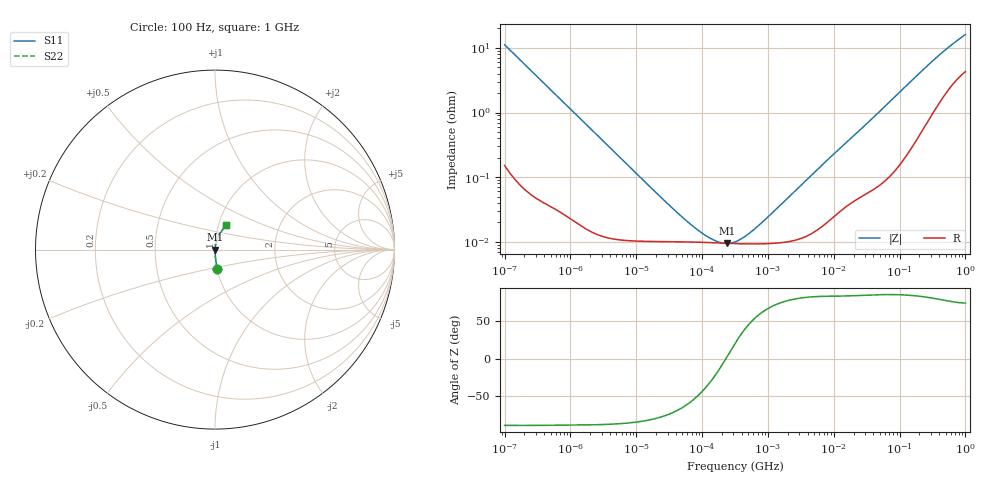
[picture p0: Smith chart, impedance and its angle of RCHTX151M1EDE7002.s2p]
! RCHTX151M1EDE7002  S-PARAMETER MODEL  (AEC-Q200 qualified)
! Model Generated by ELNA Corporation (http://www.ty-top.com)
! Version 1.0
! ELNA Control No.231201
! Copyright (c) 2023 ELNA CO.,LTD. All Rights Reserved.
! Products Name : CONDUCTIVE POLYMER HYBRID ALUMINUM ELECTROLYTIC CAPACITORS
! Characteristics :
!  Capacitance  :  150uF  ,  Rated voltage  :  16V
!  Operating Temp. Range  :  -55 to +135 degC  ,  Endurance  :  2000hr at 135 degC
!  Dimension D  :  6.3mm  ,  Dimension L  :  7.7mm
! Frequency Range : 100Hz - 1GHz
! External Node Assignments :
!  1  o---| |---o  2
# MHz S RI R 50
!Freq[MHz].  S11 Real  S11 Imag  S21 Real  S21 Imag  S12 Real  S12 Imag  S22 Real  S22 Imag
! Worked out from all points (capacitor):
!   401 points, 100 Hz to 1 GHz, reference 50 ohm
!   read as one part in series: C = 142 uF near 108 Hz
!   lowest |Z| = 9.45 mohm at 238.5 kHz (marker M1)
!   series resonance near 229.3 kHz, so ESL is about 3.4 nH
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0.0001  0.0138 -0.1101  0.9862 0.1101  0.9862 0.1101  0.0138 -0.1101
0.000113  0.0109 -0.0978  0.9891 0.0978  0.9891 0.0978  0.0109 -0.0978
0.000183  0.00442 -0.0608  0.9956 0.0608  0.9956 0.0608  0.00442 -0.0608
0.000309  0.00177 -0.0362  0.9982 0.0362  0.9982 0.0362  0.00177 -0.0362
0.001488  0.000231 -0.00763  0.9998 0.00763  0.9998 0.00763  0.000231 -0.00763
0.022131  0.000101 -0.000511  0.9999 0.000511  0.9999 0.000511  0.000101 -0.000511
0.053703  9.98e-05 -0.000202  0.9999 0.000202  0.9999 0.000202  9.98e-05 -0.000202
0.102329  9.81e-05 -9.14e-05  0.9999 9.14e-05  0.9999 9.14e-05  9.81e-05 -9.14e-05
0.135675  9.69e-05 -5.66e-05  0.9999 5.66e-05  0.9999 5.66e-05  9.69e-05 -5.66e-05
0.165959  9.6e-05 -3.42e-05  0.9999 3.42e-05  0.9999 3.42e-05  9.6e-05 -3.42e-05
0.238506  9.44e-05 4.14e-06  0.9999 -4.14e-06  0.9999 -4.14e-06  9.44e-05 4.14e-06
0.316228  9.35e-05 3.48e-05  0.9999 -3.48e-05  0.9999 -3.48e-05  9.35e-05 3.48e-05
0.356862  9.32e-05 4.88e-05  0.9999 -4.88e-05  0.9999 -4.88e-05  9.32e-05 4.88e-05
0.436516  9.29e-05 7.39e-05  0.9999 -7.39e-05  0.9999 -7.39e-05  9.29e-05 7.39e-05
0.679986  9.28e-05 0.000142  0.9999 -0.000142  0.9999 -0.000142  9.28e-05 0.000142
1.195364  9.46e-05 0.000271  0.9999 -0.000271  0.9999 -0.000271  9.46e-05 0.000271
4.704354  0.000137 0.00109  0.9999 -0.00109  0.9999 -0.00109  0.000137 0.00109
69.9842  0.00122 0.0144  0.9988 -0.0144  0.9988 -0.0144  0.00122 0.0144
169.8244  0.00454 0.0342  0.9955 -0.0342  0.9955 -0.0342  0.00454 0.0342
365.1741  0.0166 0.0682  0.9834 -0.0682  0.9834 -0.0682  0.0166 0.0682
641.9482  0.0379 0.1047  0.9621 -0.1047  0.9621 -0.1047  0.0379 0.1047
1000  0.0619 0.1397  0.9381 -0.1397  0.9381 -0.1397  0.0619 0.1397
